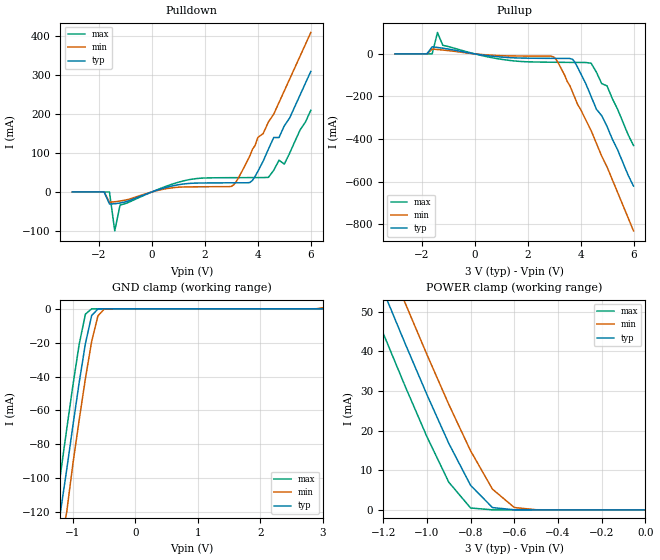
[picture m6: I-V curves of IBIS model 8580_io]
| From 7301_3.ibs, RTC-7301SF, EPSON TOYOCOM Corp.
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|   Model   8580_io
[Model]   8580_io
Model_type   I/O
Polarity   Non-Inverting
Vinl = 0.60V
Vinh = 2.40V
C_comp  8.00pF   8.00pF   8.00pF
[Temperature Range]   25   85   -40
[Voltage Range]   3.00V   2.40V   3.60V
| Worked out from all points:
|   slope of the pulldown table from 0 to 0.45 V, typ, clamps not added: 45.6 ohm
|   slope of the pullup table from 0 to 0.45 V, typ, clamps not added: 56.5 ohm
|   GND clamp passes 1 mA (typ) near -0.62 V on its own axis
|   POWER clamp passes 1 mA (typ) near -0.71 V on its own axis
[Pulldown]
|   voltage   I(typ)   I(min)   I(max)
-3V       0A         0A         0A
-1.8V     0A         0A         0A
-1.6V     -31mA      -26.4mA    0A
-1.4V     -30.34mA   -25.12mA   -100mA
-1.2V     -28.4mA    -23.34mA   -33.53mA
1.2V      20.55mA    12.84mA    28.56mA
3V        23.54mA    14.22mA    36.75mA
3.8V      29.87mA    110mA      36.94mA
4.4V      110mA      180mA      37.52mA
4.8V      140mA      230mA      81.65mA
5V        170mA      260mA      71.74mA
6V        310mA      410mA      210mA
[Pullup]
|   voltage   I(typ)   I(min)   I(max)
-3V       0A         0A         0A
-1.8V     0A         0A         0A
-1.6V     33mA       22.5mA     0A
-1.4V     29.88mA    20.28mA    100mA
-1.2V     26.37mA    17.88mA    40.3mA
0V        0A         0A         0A
3V        -21.34mA   -15.03mA   -39.49mA
3.7V      -25.71mA   -180mA     -40.25mA
4.4V      -200mA     -360mA     -44.01mA
4.8V      -290mA     -480mA     -140mA
5V        -340mA     -530mA     -150mA
6V        -620mA     -830mA     -430mA
[GND_clamp]
|   voltage   I(typ)   I(min)   I(max)
-3V       -620mA     -650mA     -600mA
-1.3V     -150mA     -170mA     -120mA
-1.2V     -120mA     -140mA     -97.79mA
-1.1V     -94.94mA   -120mA     -71.05mA
-1V       -68.74mA   -91.25mA   -45.09mA
-900mV    -43.52mA   -65.59mA   -20.92mA
-800mV    -20.48mA   -41.13mA   -3.17mA
-700mV    -3.96mA    -19.25mA   -37.79uA
-600mV    -140uA     -4.17mA    -260nA
-500mV    -2.83uA    -250uA     -1.81nA
2.8V      2.61pA     1.03uA     2pA
3V        3.01pA     590uA      2.4pA
[POWER_clamp]
|   voltage   I(typ)   I(min)   I(max)
-3V       310mA      320mA      300mA
-1.3V     68.77mA    78.97mA    58.06mA
-1.2V     55.29mA    65.5mA     44.54mA
-1.1V     42mA       52.22mA    31.24mA
-1V       29.08mA    39.19mA    18.48mA
-900mV    16.79mA    26.62mA    6.99mA
-800mV    6.18mA     14.88mA    470uA
-700mV    580uA      5.22mA     3.8uA
-600mV    13.83uA    590uA      26.22nA
-500mV    280nA      26.05uA    190pA
0V        3.01pA     26.51pA    3.6pA
[Ramp]
|variable   typ   min   max
dV/dt_r   1.62/0.78n   1.22/1.57n   2.03/0.49n
dV/dt_f   1.66/1.00n   1.29/1.88n   2.02/0.58n
R_load = 0.50k
|End   [Model] 8580_io
